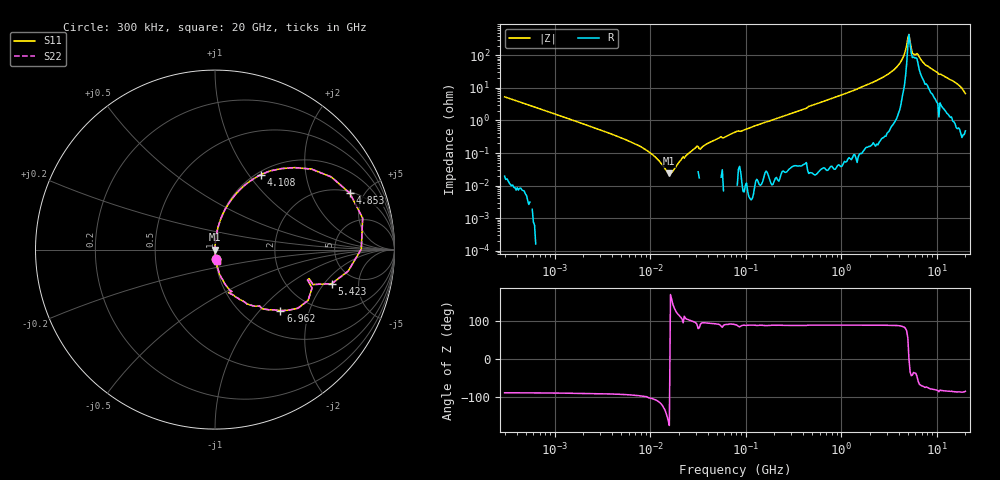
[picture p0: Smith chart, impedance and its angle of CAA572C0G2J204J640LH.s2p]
! S-Parameter Data Generated by TDK Corporation
! Copyright(C) 2022 TDK Corporation.
! All Rights Reserved.
! TDK P/N: CAA572C0G2J204J640LH (Multilayer Ceramic Chip Capacitor)
! Property: C=200nF
! Size(LxWxT): 6x5.6x6.4mm
! Model Type: s2p (Touchstone File Format Version 1.0)
! Frequency: DC=Yes Start=0.3MHz Stop=20000MHz 402points Log-sweep
! Model Generated on Apr. 15, 2022
! Port Assignments:
!  1 ---| |--- 2
! Applicable Conditions:
!  Temperature = 25 degC
!  DC Bias Voltage = 0 V
!  Small Signal Operation
! Terms and conditions regarding TDK Simulation Models
! (1)This simulation model is being provided solely for informational purposes. Please refer to the specifications of the products in terms of detailed characteristics of such products.
! (2)In no event shall TDK Corporation of any of its subsidiaries be liable for any loss or damage arising, directly or indirectly,
!  From any information contained in this simulation model, including, but not limited to loss or damages arising from any inaccuracies, omissions or errors in connection with such information.
! (3)Any and all copyrights on this simulation model are owned by TDK Corporation.
!  Duplication or redistribution of this simulation model without prior written permission from TDK Corporation is prohibited.
! (4)This simulation model is subject to any modification or change without any prior notice.
! (5)Neither TDK Corporation nor any of its subsidiaries shall make any warranty, express or implied,
!  Including but not limited to the correctness, implied warranties of merchantability and fitness for a particular purpose with respect to this simulation models.
! (6)The use of this simulation model shall be deemed to have consented to the terms and conditions hereof.
# Hz S MA R 50
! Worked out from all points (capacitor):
!   401 points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, 300 kHz to 20 GHz, reference 50 ohm
!   read as one part in series: C = 99.3 nF near 317.1 kHz
!   lowest |Z| = 24 mohm at 15.91 MHz (marker M1)
!   series resonance near 16.03 MHz, so ESL is about 990 pH
!   S11 on the Smith chart (normalised r, x): 300 kHz: 1.00, -0.11; 4.108 GHz: 1.04, +1.15; 4.853 GHz: 2.09, +3.91; 5.423 GHz: 3.41, -2.40; 6.962 GHz: 1.45, -1.31; 20 GHz: 1.01, -0.13
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300000  0.05325 -86.7  0.9984 3.1  0.9984 3.1  0.05325 -86.7
1928084  0.008169 -90.8  1 0.5  1 0.5  0.008169 -90.8
7111075  0.001861 -96.6  1 0.1  1 0.1  0.001861 -96.6
1.239169e7  0.0005793 -114.2  1 0.0  1 0.0  0.0005793 -114.2
1.590994e7  0.0002397 -176.4  1 0.0  1 0.0  0.0002397 -176.4
2.100228e7  0.000608 110.0  1 -0.0  1 -0.0  0.000608 110.0
3.013307e7  0.001484 95.6  1 -0.1  1 -0.1  0.001484 95.6
3.462121e7  0.001466 95.3  1 -0.1  1 -0.1  0.001466 95.3
7.964076e7  0.004543 90.1  1 -0.3  1 -0.3  0.004543 90.1
4.978292e8  0.02933 87.8  0.9993 -1.7  0.9993 -1.7  0.02933 87.8
1.511719e9  0.09652 84.0  0.9946 -5.5  0.9946 -5.5  0.09652 84.0
3.199522e9  0.2706 73.3  0.9581 -15.7  0.9581 -15.7  0.2706 73.3
4.10793e9  0.4896 58.6  0.854 -29.3  0.854 -29.3  0.4896 58.6
4.464803e9  0.6372 45.8  0.7196 -39.4  0.7196 -39.4  0.6372 45.8
4.85268e9  0.8144 22.7  0.4012 -51.7  0.4012 -51.7  0.8144 22.7
5.129809e9  0.8149 0.2  0.1851 -0.8  0.1851 -0.8  0.8149 0.2
5.422764e9  0.6772 -16.3  0.3982 28.5  0.3982 28.5  0.6772 -16.3
5.73245e9  0.5491 -17.1  0.5021 18.8  0.5021 18.8  0.5491 -17.1
6.962395e9  0.499 -43.0  0.7205 28.2  0.7205 28.2  0.499 -43.0
9.989315e9  0.2873 -66.7  0.9246 16.6  0.9246 16.6  0.2873 -66.7
1.601592e10  0.1395 -79.5  0.9843 8.0  0.9843 8.0  0.1395 -79.5
2e10  0.06662 -82.1  0.993 3.8  0.993 3.8  0.06662 -82.1
